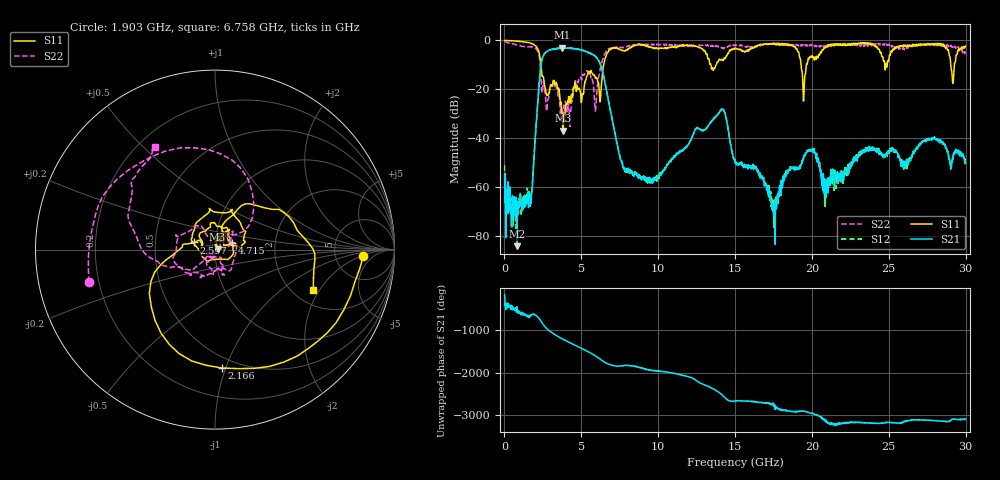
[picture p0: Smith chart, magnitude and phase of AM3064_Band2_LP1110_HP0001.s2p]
# Hz S DB R 50.0
!freq dBS11 angS11 dBS21 angS21 dBS12 angS12 dBS22 angS22
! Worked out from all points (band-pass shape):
!   1600 points, 10 MHz to 29.98 GHz, reference 50 ohm
!   highest |S21| = -3.02 dB at 3.759 GHz (marker M1); lowest = -84.2 dB at 816 MHz (marker M2)
!   |S21| within 3 dB of the highest: 2.55 GHz to 5.809 GHz (3.259 GHz wide, 78 % of centre)
!   lowest |S11| = -36.9 dB at 3.815 GHz (marker M3), VSWR 1.03, Z = 51.4 + j0.216 ohm
!   |S11| at or under -10 dB: 2.372 GHz to 6.453 GHz (4.081 GHz wide, 92.5 % of centre); 13.43 GHz to 13.77 GHz (344.5 MHz wide, 2.53 % of centre); 19.29 GHz to 19.64 GHz (348 MHz wide, 1.79 % of centre)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
!   |S22| runs from -35.2 to -0.3 dB; largest |S21 - S12| = 0.018
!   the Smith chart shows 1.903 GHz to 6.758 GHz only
!   S11 on the Smith chart (normalised r, x): 1.903 GHz: 10, -2; 2.166 GHz: 0.42, -0.97; 2.597 GHz: 0.79, +0.06; 4.715 GHz: 1.21, +0.09; 6.758 GHz: 2.53, -1.77
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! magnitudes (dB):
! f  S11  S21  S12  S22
! 10 MHz  -0.1  -54.9  -51.1  -0.3
! 816 MHz  -0.3  -84.2  -68.4  -1.9
! 1.678 GHz  -1.1  -67.9  -68.1  -2.7
! 1.903 GHz  -1.7  -49.6  -49.8  -2.8
! 2.166 GHz  -3.6  -25.3  -25.2  -4.5
! 2.597 GHz  -18.2  -5.5  -5.5  -19.7
! 3.759 GHz  -31.4  -3.0  -3.1  -30.6
! 3.815 GHz  -36.9  -3.1  -3.1  -29.8
! 4.715 GHz  -19.6  -3.6  -3.5  -17.5
! 5.015 GHz  -25.1  -3.9  -3.9  -16.1
! 5.933 GHz  -15.6  -6.7  -6.6  -28.2
! 6.758 GHz  -4.5  -24.6  -24.5  -3.6
! 7.845 GHz  -4.4  -52.7  -52.6  -2.8
! 10 GHz  -3.4  -55.8  -55.9  -1.8
! 14.14 GHz  -7.8  -28.3  -28.4  -3.0
! 15 GHz  -3.2  -50.0  -49.6  -1.9
! 17.55 GHz  -1.6  -69.7  -69.8  -1.4
! 19.47 GHz  -24.1  -47.8  -47.8  -2.3
! 19.99 GHz  -6.3  -44.8  -44.9  -1.7
! 20.91 GHz  -2.4  -63.0  -56.9  -2.5
! 25 GHz  -7.9  -45.8  -46.2  -1.7
! 29.98 GHz  -2.3  -49.9  -48.4  -4.5
